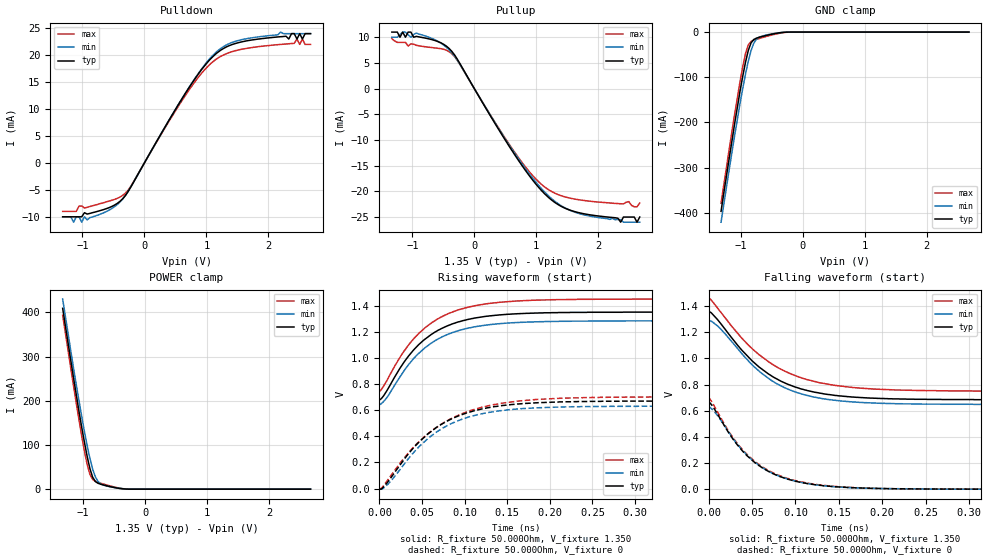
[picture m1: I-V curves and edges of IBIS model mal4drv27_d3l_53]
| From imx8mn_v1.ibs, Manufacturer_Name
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[Model] mal4drv27_d3l_53
Model_type   I/O
Polarity   Non-Inverting
Enable   Active-High
C_comp   1.534pF   1.526pF   1.541pF
C_comp_pullup   672.952fF   657.747fF   679.061fF
C_comp_pulldown 805.206fF   796.471fF   820.214fF
Vinh = 805.000mV
Vinl = 545.000mV
Vmeas = 675.000mV
Vref = 675.000mV
Rref = 50Ohms
Cref = 0pF
[Model Spec]
Vinh   805.000mV   772.000mV   855.000mV
Vinl   545.000mV   512.000mV   595.000mV
Vmeas   675.000mV   642.000mV   725.000mV
Vref   675.000mV   642.000mV   725.000mV
D_overshoot_ampl_h 0.4 NA   NA
D_overshoot_ampl_l 0.4 NA   NA
D_overshoot_area_l 110.000m NA   NA
D_overshoot_area_h 110.000m NA   NA
|[Receiver Thresholds]
|Vth = 675.000mV
|Vth_min = 642.000mV
|Vth_max = 725.000mV
|Vinh_ac = 150.000mV
|Vinh_dc = 100.000mV
|Vinl_ac = -150.000mV
|Vinl_dc = -100.000mV
|Tslew_ac = 5.000ns
|Threshold_sensitivity = 0.5
|Reference_supply Pullup_ref
[Temperature Range]   25.000   125.000   -40.000
[Voltage Range]   1.350V   1.283V   1.450V
[GND Clamp Reference]   0.00V   0.00V   0.00V
|[C Comp Corner]
|| variable   typ   min   max
|C_comp 1.541pF   1.526pF   1.534pF
|C_comp_pullup 679.061fF   657.747fF   672.952fF
|C_comp_pulldown 805.206fF   820.214fF   796.471fF
[Pulldown Reference]   0.00V   0.00V   0.00V
[POWER Clamp Reference]   1.350V   1.283V   1.450V
[Pullup Reference]   1.350V   1.283V   1.450V
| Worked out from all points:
|   slope of the pulldown table from 0 to 0.203 V, typ, clamps not added: 49.5 ohm
|   slope of the pullup table from 0 to 0.203 V, typ, clamps not added: 48.7 ohm
|   GND clamp passes 1 mA (typ) near -0.34 V on its own axis
|   POWER clamp passes 1 mA (typ) near -0.37 V on its own axis
|   rising waveform, R_fixture 50.000Ohm, V_fixture 1.350: 20-80 % time 55.9ps typ, 56ps min, 57.7ps max; typ from 0.681 V to 1.35 V
|   rising waveform, R_fixture 50.000Ohm, V_fixture 0: 20-80 % time 66.8ps typ, 64.9ps min, 74.8ps max; typ from -0.005 V to 0.67 V
|   falling waveform, R_fixture 50.000Ohm, V_fixture 1.350: 20-80 % time 66.4ps typ, 64.7ps min, 73ps max; typ from 1.35 V to 0.684 V
|   falling waveform, R_fixture 50.000Ohm, V_fixture 0: 20-80 % time 55.9ps typ, 55.8ps min, 57ps max; typ from 0.67 V to 0 V
[GND Clamp]
-1.318V   -397mA     -421mA     -379mA
-1.099V   -203mA     -229mA     -182mA
-1.011V   -130mA     -157mA     -109mA
-966.7mV  -96.76mA   -124mA     -75.62mA
-922.7mV  -66.15mA   -92.44mA   -47.23mA
-878.8mV  -40.87mA   -64.33mA   -28.32mA
-834.8mV  -24.17mA   -41.16mA   -20.75mA
-790.9mV  -16.5mA    -24.84mA   -17.97mA
-747mV    -13.39mA   -15.69mA   -16.02mA
-571.2mV  -6.876mA   -6.005mA   -9.023mA
-219.7mV  -49.34uA   -80.18uA   -119uA
2.68V     51.21nA    1.31uA     23.01nA
[Power Clamp]
-1.33V    409mA      430mA      393.3mA
-1.111V   214mA      236.6mA    194.7mA
-1.023V   140mA      164.6mA    120.2mA
-934.8mV  73.93mA    98.06mA    55.78mA
-890.9mV  46.71mA    69.56mA    33.54mA
-847mV    27.2mA     45.54mA    22.2mA
-803mV    17.25mA    27.9mA     17.76mA
-759.1mV  13.27mA    17.3mA     15.42mA
-715.2mV  11.13mA    11.9mA     13.45mA
-539.4mV  4.955mA    4.74mA     6.349mA
-275.8mV  101uA      270.7uA    142.8uA
2.668V    -162nA     -1.898uA   -65.08nA
[Pulldown]
-1.318V   -10mA      -10mA      -9mA
-1.054V   -10mA      -10mA      -8mA
-1.011V   -10mA      -11mA      -8mA
-395.5mV  -7.147mA   -7.275mA   -6.348mA
-219.7mV  -4.49mA    -4.472mA   -4.348mA
790.9mV   15.2mA     15.27mA    14.69mA
1.23V     20.92mA    21.24mA    19.77mA
1.714V    22.79mA    23.19mA    21.39mA
2.329V    23mA       24mA       22.12mA
2.373V    24mA       24mA       22.16mA
2.461V    23mA       24mA       23mA
2.68V     24mA       24mA       22mA
[Pullup]
-1.33V    11mA       10mA       9.724mA
-934.8mV  10.17mA    10.82mA    8.425mA
-407.6mV  7.821mA    7.564mA    7.201mA
-275.8mV  5.756mA    5.567mA    5.534mA
734.8mV   -14.37mA   -14.05mA   -13.81mA
1.262V    -21.83mA   -21.58mA   -20.13mA
1.658V    -24.07mA   -24.2mA    -21.58mA
2.361V    -26mA      -25.52mA   -22.41mA
2.405V    -25mA      -26mA      -22.44mA
2.58V     -25mA      -26mA      -23mA
2.624V    -26mA      -26mA      -23mA
2.668V    -25mA      -26mA      -22.28mA
[Ramp]
R_load=50.000Ohm
dV/dt_r   400.800mV/62.000ps  379.498mV/61.500ps  420.900mV/67.000ps
dV/dt_f   400.800mV/62.000ps  379.498mV/60.500ps  420.900mV/65.500ps
[Rising waveform]
R_fixture=50.000Ohm
V_fixture=1.350
V_fixture_min=1.283
V_fixture_max=1.450
0s        681mV      644mV      748mV
2ps       687mV      649mV      756mV
8ps       740mV      690mV      819mV
29ps      969mV      903mV      1.053V
48ps      1.113V     1.047V     1.199V
73ps      1.225V     1.159V     1.314V
106ps     1.297V     1.23V      1.391V
140ps     1.328V     1.261V     1.425V
208ps     1.346V     1.279V     1.446V
470ps     1.35V      1.283V     1.45V
[Rising waveform]
R_fixture=50.000Ohm
V_fixture=0
0s        -4.835mV   -4.338mV   -231.3uV
2ps       -4.835mV   -4.338mV   -231.3uV
10ps      52.2mV     33.48mV    68.24mV
37ps      290mV      252mV      296mV
59ps      430mV      394mV      430mV
91ps      551mV      516mV      556mV
128ps     619mV      582mV      634mV
162ps     647mV      609mV      669mV
212ps     663mV      624mV      691mV
471ps     670mV      630mV      702mV
[Falling waveform]
R_fixture=50.000Ohm
V_fixture=1.350
V_fixture_min=1.283
V_fixture_max=1.450
0s        1.353V     1.285V     1.453V
2ps       1.353V     1.285V     1.453V
13ps      1.273V     1.23V      1.361V
40ps      1.049V     1.022V     1.141V
64ps      903mV      870mV      997mV
94ps      795mV      757mV      883mV
128ps     734mV      696mV      813mV
167ps     704mV      666mV      776mV
215ps     690mV      653mV      758mV
471ps     684mV      648mV      749mV
[Falling waveform]
R_fixture=50.000Ohm
V_fixture=0
0s        670mV      633mV      702mV
9ps       588mV      574mV      605mV
26ps      402mV      407mV      413mV
45ps      251mV      254mV      260mV
56ps      189mV      191mV      198mV
72ps      126mV      126mV      132mV
103ps     56.25mV    56.13mV    60.48mV
143ps     19.71mV    19.59mV    21.78mV
188ps     6.302mV    6.008mV    6.782mV
469ps     19.78uV    25.75uV    20.37uV
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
